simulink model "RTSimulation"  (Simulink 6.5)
settings: Solver=FixedStepDiscrete  StartTime=0.0  StopTime=inf  RelTol=1e-3
PreLoadFcn:
  | initialize
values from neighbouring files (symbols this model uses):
  actParams = [	bulkModulus   * pressCanon    [Copy of initialize.m]    (also in initialize.m = [bulkModulus	* pressCanon,)
  displFreq = inf    [initialize.m]
  flowCanon = 1.666667e+04    (= 16666.67)    [Copy of initialize.m]    (also in initialize.m)
  forceCanon = 1    [Copy of initialize.m]    (also in initialize.m)
  forceFreq = inf    [initialize.m]
  friction = 5			 				* 0.155000	 				* 0.00444822 				* area1    (= 2.71252900422)    [initialize.m]
  fsamp = 1 / samplePeriod    (= 1024)    [Copy of initialize.m]    (also in initialize.m; rampth.m = 1 / deltaT; randth.m = 1 / deltaT; rspect.m = 1.0 / tsamp)
  gasConstant = 1.8    [Copy of initialize.m]    (also in initialize.m)
  lengthCanon = 1    [Copy of initialize.m]    (also in initialize.m)
  massCanon = 1e-06    [Copy of initialize.m]    (also in initialize.m)
  maxDispl = ( (stroke2 + endLength2) * lengthCanon)'    [Copy of initialize.m]    (also in initialize.m = 576.2)
  maxOilVolume = volume * (1 - (precharge/supplyPress)^(1/gasConstant))    (= 211.391477114)    [Copy of initialize.m]    (also in initialize.m)
  maxVeloc = ( (maxFlow' * flowCanon ./ (area1 * areaCanon)) / velocCanon)'    [Copy of initialize.m]    (also in initialize.m = (maxFlow * flowCanon / (area1 * areaCanon)) / velocCanon; rampth.m = 2 * maxDispl / (nVeloc * deltaT))
  minDispl = (-(stroke1 + endLength1) * lengthCanon)'    [Copy of initialize.m]    (also in initialize.m = -576.2)
  minVeloc = (-(maxFlow' * flowCanon ./ (area2 * areaCanon)) / velocCanon)'    [Copy of initialize.m]    (also in initialize.m = -(maxFlow * flowCanon / (area2 * areaCanon)) / velocCanon)
  nAct = 5    [Copy of initialize.m]    (also in initialize.m = 1)
  nAdcU = 6    [Copy of initialize.m]    (also in initialize.m = 5)
  nDout = 4    [Copy of initialize.m]    (also in initialize.m)
  nDucU = 2    [Copy of initialize.m]    (also in initialize.m)
  nEncU = 3    [Copy of initialize.m]    (also in initialize.m)
  node = completenodestruct(node)    [Copy of initialize.m]    (also in initialize.m)
  precharge = 3000		 				* 6.894757e-03    (= 20.684271)    [Copy of initialize.m]    (also in initialize.m)
  pumpFlow = 1e20    (= 1e+20)    [Copy of initialize.m]    (also in initialize.m)
  returnPress = 3			 				* 0.1    (= 0.3)    [Copy of initialize.m]    (also in initialize.m)
  samplePeriod = controlPeriod/upsampleFactor    (= 0.0009765625)    [Copy of initialize.m]    (also in initialize.m; viewer.m = eval(getHeaderValue(header, 'DELTA_T')))
  springCanon = 1    [Copy of initialize.m]    (also in initialize.m)
  supplyPress = 280		 				* 0.1    (= 28)    [Copy of initialize.m]    (also in initialize.m)
  velocCanon = 1    [Copy of initialize.m]    (also in initialize.m)
  volume = 15.15		 				+ (  45		 				    * 2		 				   + 30		 				    * 6 )	 				* 5    (= 1365.15)    [Copy of initialize.m]    (also in initialize.m; quake.m = volume / 231.0)
  volumeCanon = 1e+06    (= 1000000)    [Copy of initialize.m]    (also in initialize.m)
  yieldDispl = 1.0    (= 1)    [initialize.m]
undefined symbols (not defined in the file or in its folder): DiscIntNeverNeededParam, dpforceFreq, mass, spring, staticForce
libraries: xpclib x5
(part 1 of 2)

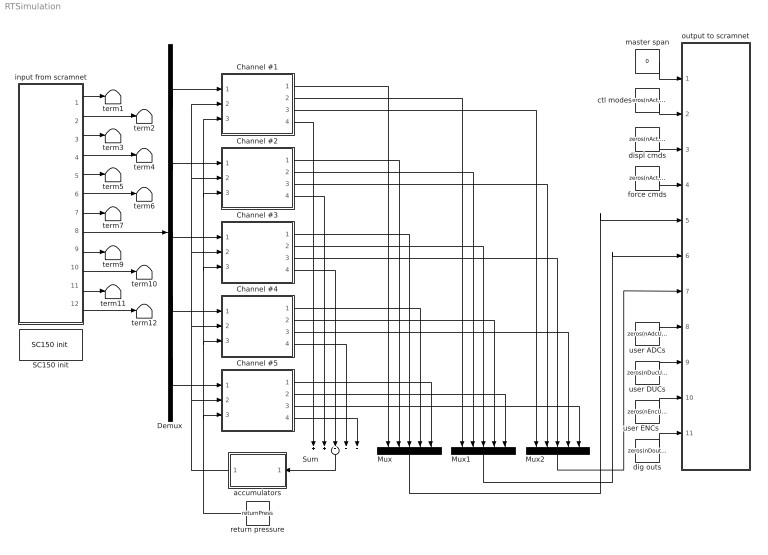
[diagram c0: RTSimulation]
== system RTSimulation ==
  Channel #1 : Subsystem  mask{id=1}
      mask prompts: id "Channel ID"
  Channel #2 : Subsystem  mask{id=2}
      mask prompts: id "Channel ID"
  Channel #3 : Subsystem  mask{id=3}
      mask prompts: id "Channel ID"
  Channel #4 : Subsystem  mask{id=4}
      mask prompts: id "Channel ID"
  Channel #5 : Subsystem  mask{id=5}
      mask prompts: id "Channel ID"
  Demux : Demux  Outputs=nAct
  Mux : Mux  Orientation=down  Inputs=nAct
  Mux1 : Mux  Orientation=down  Inputs=nAct
  Mux2 : Mux  Orientation=down  Inputs=nAct
  SC150 init : xpclib/Shared Memory/Systran/SC150 init   node=node  pci=-1
  Sum : Sum  Orientation=down  Inputs=+++++
  accumulators : Subsystem  Orientation=left
  ctl modes : Constant  Value=zeros(nAct, 1)  OutDataType=sfix(16)  ConRadixGroup=Use specified scaling  OutScaling=2^0  SampleTime=inf  FramePeriod=inf
  dig outs : Constant  Value=zeros(nDout, 1)  OutDataTypeMode=uint32  OutDataType=sfix(16)  ConRadixGroup=Use specified scaling  OutScaling=2^0  SampleTime=inf  FramePeriod=inf
  displ cmds : Constant  Value=zeros(nAct, 1)  OutDataType=sfix(16)  ConRadixGroup=Use specified scaling  OutScaling=2^0  SampleTime=inf  FramePeriod=inf
  force cmds : Constant  Value=zeros(nAct, 1)  OutDataType=sfix(16)  ConRadixGroup=Use specified scaling  OutScaling=2^0  SampleTime=inf  FramePeriod=inf
  input from scramnet : Subsystem
  master span : Constant  Value=0  OutDataType=sfix(16)  ConRadixGroup=Use specified scaling  OutScaling=2^0  SampleTime=inf  FramePeriod=inf
  output to scramnet : Subsystem
  return pressure : Constant  Orientation=left  Value=returnPress  OutDataType=sfix(16)  ConRadixGroup=Use specified scaling  OutScaling=2^0  SampleTime=inf  FramePeriod=inf
  term{1..7,9..12} (11 alike) : Terminator
  user ADCs : Constant  Value=zeros(nAdcU, 1)  OutDataType=sfix(16)  ConRadixGroup=Use specified scaling  OutScaling=2^0  SampleTime=inf  FramePeriod=inf
  user DUCs : Constant  Value=zeros(nDucU, 1)  OutDataType=sfix(16)  ConRadixGroup=Use specified scaling  OutScaling=2^0  SampleTime=inf  FramePeriod=inf
  user ENCs : Constant  Value=zeros(nEncU, 1)  OutDataType=sfix(16)  ConRadixGroup=Use specified scaling  OutScaling=2^0  SampleTime=inf  FramePeriod=inf
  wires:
  input from scramnet/6(force fbks) -> term6/1
  input from scramnet/10(user ducs) -> term10/1
  input from scramnet/12(dig inps) -> term12/1
  input from scramnet/4(force cmds) -> term4/1
  input from scramnet/5(displ fbks) -> term5/1
  input from scramnet/7(dpforce fbks) -> term7/1
  input from scramnet/9(user adcs) -> term9/1
  input from scramnet/11(user encs) -> term11/1
  input from scramnet/1(master span) -> term1/1
  input from scramnet/2(ctl modes) -> term2/1
  input from scramnet/3(displ cmds) -> term3/1
  master span/1 -> output to scramnet/1(master span)
  ctl modes/1 -> output to scramnet/2(ctl modes)
  displ cmds/1 -> output to scramnet/3(displ cmds)
  force cmds/1 -> output to scramnet/4(force cmds)
  user ADCs/1 -> output to scramnet/8(user adcs)
  user DUCs/1 -> output to scramnet/9(user ducs)
  user ENCs/1 -> output to scramnet/10(user encs)
  dig outs/1 -> output to scramnet/11(dig outs)
  Channel #1/4(flow) -> Sum/1
  Channel #2/4(flow) -> Sum/2
  Channel #3/4(flow) -> Sum/3
  Sum/1 -> accumulators/1(flow)
  Channel #4/4(flow) -> Sum/4
  Channel #5/4(flow) -> Sum/5
  Channel #1/1(displ) -> Mux/1
  Channel #2/1(displ) -> Mux/2
  Channel #3/1(displ) -> Mux/3
  Channel #4/1(displ) -> Mux/4
  Channel #5/1(displ) -> Mux/5
  Channel #1/2(force) -> Mux1/1
  Channel #2/2(force) -> Mux1/2
  Channel #3/2(force) -> Mux1/3
  Channel #4/2(force) -> Mux1/4
  Channel #5/2(force) -> Mux1/5
  Channel #1/3(dpforce) -> Mux2/1
  Channel #2/3(dpforce) -> Mux2/2
  Channel #3/3(dpforce) -> Mux2/3
  Channel #4/3(dpforce) -> Mux2/4
  Channel #5/3(dpforce) -> Mux2/5
  Mux/1 -> output to scramnet/5(displ fbks)
  Mux1/1 -> output to scramnet/6(force fbks)
  Mux2/1 -> output to scramnet/7(dpforce fbks)
  input from scramnet/8(valve cmds) -> Demux/1
  Demux/1 -> Channel #1/1(valve cmd)
  Demux/2 -> Channel #2/1(valve cmd)
  Demux/3 -> Channel #3/1(valve cmd)
  Demux/4 -> Channel #4/1(valve cmd)
  Demux/5 -> Channel #5/1(valve cmd)
  accumulators/1(press) -> Channel #2/2(spl press), Channel #1/2(spl press), Channel #3/2(spl press), Channel #4/2(spl press), Channel #5/2(spl press)
  return pressure/1 -> Channel #2/3(rtn press), Channel #1/3(rtn press), Channel #3/3(rtn press), Channel #4/3(rtn press), Channel #5/3(rtn press)

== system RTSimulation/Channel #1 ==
  valve cmd : Inport
  spl press : Inport  Port=2
  rtn press : Inport  Port=3
  displ cond filter : Subsystem  mask{freq3dB=displFreq(id), fsamp=fsamp}
      mask prompts: freq3dB "3 dB cutoff frequency (inf, 500, 300, 100, 50 Hz)"; fsamp "Sampling frequency (Hz)"
      mask init:
      | if isempty(freq3dB)
      | 	freq3dB = fsamp;
      | elseif freq3dB == 500
      | 	freq3dB = 485;
      | elseif freq3dB == 300
      | 	freq3dB = 204.9;
      | elseif freq3dB == 100
      | 	freq3dB = 56.5;
      | elseif freq3dB == 50
      | 	freq3dB = 27.8;
      | else
      | 	freq3dB = fsamp;
      | end
      | if freq3dB > fsamp/2
      | 	a = [1];
      | 	b = [1];
      | else
      | 	[b, a] = ellip(4, 0.001, 60.0, 2*freq3dB/fsamp);
      | end
  dpforce cond filter : Subsystem  mask{freq3dB=dpforceFreq(id), fsamp=fsamp}
      mask prompts: freq3dB "3 dB cutoff frequency (inf, 500, 300, 100, 50 Hz)"; fsamp "Sampling frequency (Hz)"
      mask init:
      | if isempty(freq3dB)
      | 	freq3dB = fsamp;
      | elseif freq3dB == 500
      | 	freq3dB = 485;
      | elseif freq3dB == 300
      | 	freq3dB = 204.9;
      | elseif freq3dB == 100
      | 	freq3dB = 56.5;
      | elseif freq3dB == 50
      | 	freq3dB = 27.8;
      | else
      | 	freq3dB = fsamp;
      | end
      | if freq3dB > fsamp/2
      | 	a = [1];
      | 	b = [1];
      | else
      | 	[b, a] = ellip(4, 0.001, 60.0, 2*freq3dB/fsamp);
      | end
  force cond filter : Subsystem  mask{freq3dB=forceFreq((id)), fsamp=fsamp}
      mask prompts: freq3dB "3 dB cutoff frequency (inf, 500, 300, 100, 50 Hz)"; fsamp "Sampling frequency (Hz)"
      mask init:
      | if isempty(freq3dB)
      | 	freq3dB = fsamp;
      | elseif freq3dB == 500
      | 	freq3dB = 485;
      | elseif freq3dB == 300
      | 	freq3dB = 204.9;
      | elseif freq3dB == 100
      | 	freq3dB = 56.5;
      | elseif freq3dB == 50
      | 	freq3dB = 27.8;
      | else
      | 	freq3dB = fsamp;
      | end
      | if freq3dB > fsamp/2
      | 	a = [1];
      | 	b = [1];
      | else
      | 	[b, a] = ellip(4, 0.001, 60.0, 2*freq3dB/fsamp);
      | end
  payload : Subsystem
  servovalve & actuator : Subsystem  mask(Actuator){params=actParams(:,id)}
      mask prompts: params "Parameter vector"
  displ : Outport
  force : Outport  Port=2
  dpforce : Outport  Port=3
  flow : Outport  Port=4
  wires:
  dpforce cond filter/1(out) -> dpforce/1
  force cond filter/1(out) -> force/1
  displ cond filter/1(out) -> displ/1
  servovalve & actuator/1(force) -> payload/1(force), dpforce cond filter/1(inp), force cond filter/1(inp)
  servovalve & actuator/2(flow) -> flow/1
  spl press/1 -> servovalve & actuator/4(spl press)
  rtn press/1 -> servovalve & actuator/5(rtn press)
  valve cmd/1 -> servovalve & actuator/1(cmd)
  payload/1(displ) -> servovalve & actuator/2(displ), displ cond filter/1(inp)
  payload/2(veloc) -> servovalve & actuator/3(veloc)

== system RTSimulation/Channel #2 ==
  valve cmd : Inport
  spl press : Inport  Port=2
  rtn press : Inport  Port=3
  displ cond filter : Subsystem  mask{freq3dB=displFreq(id), fsamp=fsamp}
      mask prompts: freq3dB "3 dB cutoff frequency (inf, 500, 300, 100, 50 Hz)"; fsamp "Sampling frequency (Hz)"
      mask init:
      | if isempty(freq3dB)
      | 	freq3dB = fsamp;
      | elseif freq3dB == 500
      | 	freq3dB = 485;
      | elseif freq3dB == 300
      | 	freq3dB = 204.9;
      | elseif freq3dB == 100
      | 	freq3dB = 56.5;
      | elseif freq3dB == 50
      | 	freq3dB = 27.8;
      | else
      | 	freq3dB = fsamp;
      | end
      | if freq3dB > fsamp/2
      | 	a = [1];
      | 	b = [1];
      | else
      | 	[b, a] = ellip(4, 0.001, 60.0, 2*freq3dB/fsamp);
      | end
  dpforce cond filter : Subsystem  mask{freq3dB=dpforceFreq(id), fsamp=fsamp}
      mask prompts: freq3dB "3 dB cutoff frequency (inf, 500, 300, 100, 50 Hz)"; fsamp "Sampling frequency (Hz)"
      mask init:
      | if isempty(freq3dB)
      | 	freq3dB = fsamp;
      | elseif freq3dB == 500
      | 	freq3dB = 485;
      | elseif freq3dB == 300
      | 	freq3dB = 204.9;
      | elseif freq3dB == 100
      | 	freq3dB = 56.5;
      | elseif freq3dB == 50
      | 	freq3dB = 27.8;
      | else
      | 	freq3dB = fsamp;
      | end
      | if freq3dB > fsamp/2
      | 	a = [1];
      | 	b = [1];
      | else
      | 	[b, a] = ellip(4, 0.001, 60.0, 2*freq3dB/fsamp);
      | end
  force cond filter : Subsystem  mask{freq3dB=forceFreq((id)), fsamp=fsamp}
      mask prompts: freq3dB "3 dB cutoff frequency (inf, 500, 300, 100, 50 Hz)"; fsamp "Sampling frequency (Hz)"
      mask init:
      | if isempty(freq3dB)
      | 	freq3dB = fsamp;
      | elseif freq3dB == 500
      | 	freq3dB = 485;
      | elseif freq3dB == 300
      | 	freq3dB = 204.9;
      | elseif freq3dB == 100
      | 	freq3dB = 56.5;
      | elseif freq3dB == 50
      | 	freq3dB = 27.8;
      | else
      | 	freq3dB = fsamp;
      | end
      | if freq3dB > fsamp/2
      | 	a = [1];
      | 	b = [1];
      | else
      | 	[b, a] = ellip(4, 0.001, 60.0, 2*freq3dB/fsamp);
      | end
  payload : Subsystem
  servovalve & actuator : Subsystem  mask(Actuator){params=actParams(:,id)}
      mask prompts: params "Parameter vector"
  displ : Outport
  force : Outport  Port=2
  dpforce : Outport  Port=3
  flow : Outport  Port=4
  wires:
  payload/2(veloc) -> servovalve & actuator/3(veloc)
  payload/1(displ) -> displ cond filter/1(inp), servovalve & actuator/2(displ)
  valve cmd/1 -> servovalve & actuator/1(cmd)
  rtn press/1 -> servovalve & actuator/5(rtn press)
  spl press/1 -> servovalve & actuator/4(spl press)
  servovalve & actuator/2(flow) -> flow/1
  servovalve & actuator/1(force) -> force cond filter/1(inp), dpforce cond filter/1(inp), payload/1(force)
  displ cond filter/1(out) -> displ/1
  force cond filter/1(out) -> force/1
  dpforce cond filter/1(out) -> dpforce/1

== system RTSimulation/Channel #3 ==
  valve cmd : Inport
  spl press : Inport  Port=2
  rtn press : Inport  Port=3
  displ cond filter : Subsystem  mask{freq3dB=displFreq(id), fsamp=fsamp}
      mask prompts: freq3dB "3 dB cutoff frequency (inf, 500, 300, 100, 50 Hz)"; fsamp "Sampling frequency (Hz)"
      mask init:
      | if isempty(freq3dB)
      | 	freq3dB = fsamp;
      | elseif freq3dB == 500
      | 	freq3dB = 485;
      | elseif freq3dB == 300
      | 	freq3dB = 204.9;
      | elseif freq3dB == 100
      | 	freq3dB = 56.5;
      | elseif freq3dB == 50
      | 	freq3dB = 27.8;
      | else
      | 	freq3dB = fsamp;
      | end
      | if freq3dB > fsamp/2
      | 	a = [1];
      | 	b = [1];
      | else
      | 	[b, a] = ellip(4, 0.001, 60.0, 2*freq3dB/fsamp);
      | end
  dpforce cond filter : Subsystem  mask{freq3dB=dpforceFreq(id), fsamp=fsamp}
      mask prompts: freq3dB "3 dB cutoff frequency (inf, 500, 300, 100, 50 Hz)"; fsamp "Sampling frequency (Hz)"
      mask init:
      | if isempty(freq3dB)
      | 	freq3dB = fsamp;
      | elseif freq3dB == 500
      | 	freq3dB = 485;
      | elseif freq3dB == 300
      | 	freq3dB = 204.9;
      | elseif freq3dB == 100
      | 	freq3dB = 56.5;
      | elseif freq3dB == 50
      | 	freq3dB = 27.8;
      | else
      | 	freq3dB = fsamp;
      | end
      | if freq3dB > fsamp/2
      | 	a = [1];
      | 	b = [1];
      | else
      | 	[b, a] = ellip(4, 0.001, 60.0, 2*freq3dB/fsamp);
      | end
  force cond filter : Subsystem  mask{freq3dB=forceFreq((id)), fsamp=fsamp}
      mask prompts: freq3dB "3 dB cutoff frequency (inf, 500, 300, 100, 50 Hz)"; fsamp "Sampling frequency (Hz)"
      mask init:
      | if isempty(freq3dB)
      | 	freq3dB = fsamp;
      | elseif freq3dB == 500
      | 	freq3dB = 485;
      | elseif freq3dB == 300
      | 	freq3dB = 204.9;
      | elseif freq3dB == 100
      | 	freq3dB = 56.5;
      | elseif freq3dB == 50
      | 	freq3dB = 27.8;
      | else
      | 	freq3dB = fsamp;
      | end
      | if freq3dB > fsamp/2
      | 	a = [1];
      | 	b = [1];
      | else
      | 	[b, a] = ellip(4, 0.001, 60.0, 2*freq3dB/fsamp);
      | end
  payload : Subsystem
  servovalve & actuator : Subsystem  mask(Actuator){params=actParams(:,id)}
      mask prompts: params "Parameter vector"
  displ : Outport
  force : Outport  Port=2
  dpforce : Outport  Port=3
  flow : Outport  Port=4
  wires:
  dpforce cond filter/1(out) -> dpforce/1
  force cond filter/1(out) -> force/1
  displ cond filter/1(out) -> displ/1
  servovalve & actuator/1(force) -> payload/1(force), dpforce cond filter/1(inp), force cond filter/1(inp)
  servovalve & actuator/2(flow) -> flow/1
  spl press/1 -> servovalve & actuator/4(spl press)
  rtn press/1 -> servovalve & actuator/5(rtn press)
  valve cmd/1 -> servovalve & actuator/1(cmd)
  payload/1(displ) -> servovalve & actuator/2(displ), displ cond filter/1(inp)
  payload/2(veloc) -> servovalve & actuator/3(veloc)

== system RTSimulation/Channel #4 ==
  valve cmd : Inport
  spl press : Inport  Port=2
  rtn press : Inport  Port=3
  displ cond filter : Subsystem  mask{freq3dB=displFreq(id), fsamp=fsamp}
      mask prompts: freq3dB "3 dB cutoff frequency (inf, 500, 300, 100, 50 Hz)"; fsamp "Sampling frequency (Hz)"
      mask init:
      | if isempty(freq3dB)
      | 	freq3dB = fsamp;
      | elseif freq3dB == 500
      | 	freq3dB = 485;
      | elseif freq3dB == 300
      | 	freq3dB = 204.9;
      | elseif freq3dB == 100
      | 	freq3dB = 56.5;
      | elseif freq3dB == 50
      | 	freq3dB = 27.8;
      | else
      | 	freq3dB = fsamp;
      | end
      | if freq3dB > fsamp/2
      | 	a = [1];
      | 	b = [1];
      | else
      | 	[b, a] = ellip(4, 0.001, 60.0, 2*freq3dB/fsamp);
      | end
  dpforce cond filter : Subsystem  mask{freq3dB=dpforceFreq(id), fsamp=fsamp}
      mask prompts: freq3dB "3 dB cutoff frequency (inf, 500, 300, 100, 50 Hz)"; fsamp "Sampling frequency (Hz)"
      mask init:
      | if isempty(freq3dB)
      | 	freq3dB = fsamp;
      | elseif freq3dB == 500
      | 	freq3dB = 485;
      | elseif freq3dB == 300
      | 	freq3dB = 204.9;
      | elseif freq3dB == 100
      | 	freq3dB = 56.5;
      | elseif freq3dB == 50
      | 	freq3dB = 27.8;
      | else
      | 	freq3dB = fsamp;
      | end
      | if freq3dB > fsamp/2
      | 	a = [1];
      | 	b = [1];
      | else
      | 	[b, a] = ellip(4, 0.001, 60.0, 2*freq3dB/fsamp);
      | end
  force cond filter : Subsystem  mask{freq3dB=forceFreq((id)), fsamp=fsamp}
      mask prompts: freq3dB "3 dB cutoff frequency (inf, 500, 300, 100, 50 Hz)"; fsamp "Sampling frequency (Hz)"
      mask init:
      | if isempty(freq3dB)
      | 	freq3dB = fsamp;
      | elseif freq3dB == 500
      | 	freq3dB = 485;
      | elseif freq3dB == 300
      | 	freq3dB = 204.9;
      | elseif freq3dB == 100
      | 	freq3dB = 56.5;
      | elseif freq3dB == 50
      | 	freq3dB = 27.8;
      | else
      | 	freq3dB = fsamp;
      | end
      | if freq3dB > fsamp/2
      | 	a = [1];
      | 	b = [1];
      | else
      | 	[b, a] = ellip(4, 0.001, 60.0, 2*freq3dB/fsamp);
      | end
  payload : Subsystem
  servovalve & actuator : Subsystem  mask(Actuator){params=actParams(:,id)}
      mask prompts: params "Parameter vector"
  displ : Outport
  force : Outport  Port=2
  dpforce : Outport  Port=3
  flow : Outport  Port=4
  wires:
  payload/2(veloc) -> servovalve & actuator/3(veloc)
  payload/1(displ) -> displ cond filter/1(inp), servovalve & actuator/2(displ)
  valve cmd/1 -> servovalve & actuator/1(cmd)
  rtn press/1 -> servovalve & actuator/5(rtn press)
  spl press/1 -> servovalve & actuator/4(spl press)
  servovalve & actuator/2(flow) -> flow/1
  servovalve & actuator/1(force) -> force cond filter/1(inp), dpforce cond filter/1(inp), payload/1(force)
  displ cond filter/1(out) -> displ/1
  force cond filter/1(out) -> force/1
  dpforce cond filter/1(out) -> dpforce/1

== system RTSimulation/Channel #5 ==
  valve cmd : Inport
  spl press : Inport  Port=2
  rtn press : Inport  Port=3
  displ cond filter : Subsystem  mask{freq3dB=displFreq(id), fsamp=fsamp}
      mask prompts: freq3dB "3 dB cutoff frequency (inf, 500, 300, 100, 50 Hz)"; fsamp "Sampling frequency (Hz)"
      mask init:
      | if isempty(freq3dB)
      | 	freq3dB = fsamp;
      | elseif freq3dB == 500
      | 	freq3dB = 485;
      | elseif freq3dB == 300
      | 	freq3dB = 204.9;
      | elseif freq3dB == 100
      | 	freq3dB = 56.5;
      | elseif freq3dB == 50
      | 	freq3dB = 27.8;
      | else
      | 	freq3dB = fsamp;
      | end
      | if freq3dB > fsamp/2
      | 	a = [1];
      | 	b = [1];
      | else
      | 	[b, a] = ellip(4, 0.001, 60.0, 2*freq3dB/fsamp);
      | end
  dpforce cond filter : Subsystem  mask{freq3dB=dpforceFreq(id), fsamp=fsamp}
      mask prompts: freq3dB "3 dB cutoff frequency (inf, 500, 300, 100, 50 Hz)"; fsamp "Sampling frequency (Hz)"
      mask init:
      | if isempty(freq3dB)
      | 	freq3dB = fsamp;
      | elseif freq3dB == 500
      | 	freq3dB = 485;
      | elseif freq3dB == 300
      | 	freq3dB = 204.9;
      | elseif freq3dB == 100
      | 	freq3dB = 56.5;
      | elseif freq3dB == 50
      | 	freq3dB = 27.8;
      | else
      | 	freq3dB = fsamp;
      | end
      | if freq3dB > fsamp/2
      | 	a = [1];
      | 	b = [1];
      | else
      | 	[b, a] = ellip(4, 0.001, 60.0, 2*freq3dB/fsamp);
      | end
  force cond filter : Subsystem  mask{freq3dB=forceFreq((id)), fsamp=fsamp}
      mask prompts: freq3dB "3 dB cutoff frequency (inf, 500, 300, 100, 50 Hz)"; fsamp "Sampling frequency (Hz)"
      mask init:
      | if isempty(freq3dB)
      | 	freq3dB = fsamp;
      | elseif freq3dB == 500
      | 	freq3dB = 485;
      | elseif freq3dB == 300
      | 	freq3dB = 204.9;
      | elseif freq3dB == 100
      | 	freq3dB = 56.5;
      | elseif freq3dB == 50
      | 	freq3dB = 27.8;
      | else
      | 	freq3dB = fsamp;
      | end
      | if freq3dB > fsamp/2
      | 	a = [1];
      | 	b = [1];
      | else
      | 	[b, a] = ellip(4, 0.001, 60.0, 2*freq3dB/fsamp);
      | end
  payload : Subsystem
  servovalve & actuator : Subsystem  mask(Actuator){params=actParams(:,id)}
      mask prompts: params "Parameter vector"
  displ : Outport
  force : Outport  Port=2
  dpforce : Outport  Port=3
  flow : Outport  Port=4
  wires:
  dpforce cond filter/1(out) -> dpforce/1
  force cond filter/1(out) -> force/1
  displ cond filter/1(out) -> displ/1
  servovalve & actuator/1(force) -> payload/1(force), dpforce cond filter/1(inp), force cond filter/1(inp)
  servovalve & actuator/2(flow) -> flow/1
  spl press/1 -> servovalve & actuator/4(spl press)
  rtn press/1 -> servovalve & actuator/5(rtn press)
  valve cmd/1 -> servovalve & actuator/1(cmd)
  payload/1(displ) -> servovalve & actuator/2(displ), displ cond filter/1(inp)
  payload/2(veloc) -> servovalve & actuator/3(veloc)

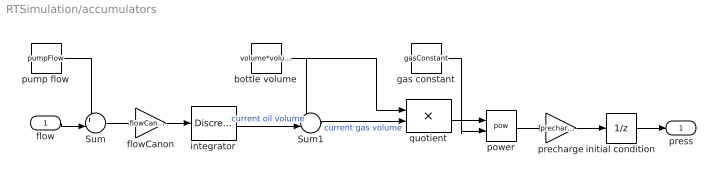
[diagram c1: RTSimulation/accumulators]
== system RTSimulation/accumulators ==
  flow : Inport
  Sum : Sum  Inputs=+-|
  Sum1 : Sum  Inputs=+-|
  bottle volume : Constant  Value=volume*volumeCanon  OutDataType=sfix(16)  ConRadixGroup=Use specified scaling  OutScaling=2^0  SampleTime=inf  FramePeriod=inf
  flowCanon : Gain  Gain=flowCanon
  gas constant : Constant  Value=gasConstant  OutDataType=sfix(16)  ConRadixGroup=Use specified scaling  OutScaling=2^0  SampleTime=inf  FramePeriod=inf
  initial condition : UnitDelay  X0=supplyPress  SampleTime=-1
  integrator : DiscreteIntegrator  InitialCondition=maxOilVolume*volumeCanon  SampleTime=-1  LimitOutput=on  UpperSaturationLimit=maxOilVolume*volumeCanon  LowerSaturationLimit=0  ICPrevOutput=DiscIntNeverNeededParam  ICPrevScaledInput=DiscIntNeverNeededParam
  power : Math  Operator=pow
  precharge : Gain  Gain=precharge
  pump flow : Constant  Value=pumpFlow  OutDataType=sfix(16)  ConRadixGroup=Use specified scaling  OutScaling=2^0  SampleTime=inf  FramePeriod=inf
  quotient : Product  Inputs=*/
  press : Outport
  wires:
  pump flow/1 -> Sum/1
  Sum/1 -> flowCanon/1
  bottle volume/1 -> Sum1/1, quotient/1
  gas constant/1 -> power/2
  power/1 -> precharge/1
  precharge/1 -> initial condition/1
  Sum1/1 -> quotient/2  "current gas volume"
  quotient/1 -> power/1
  integrator/1 -> Sum1/2  "current oil volume"
  flow/1 -> Sum/2
  flowCanon/1 -> integrator/1
  initial condition/1 -> press/1

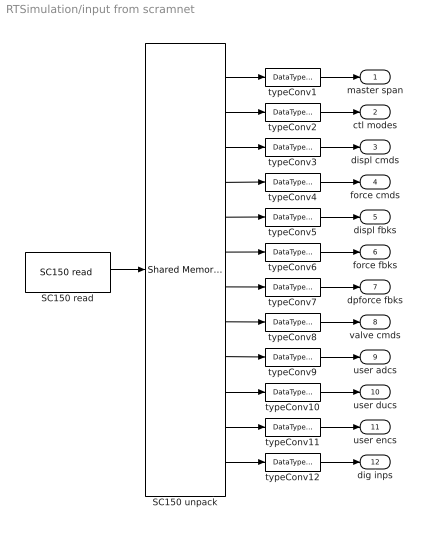
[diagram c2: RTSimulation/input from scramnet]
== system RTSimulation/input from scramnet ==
  SC150 read : xpclib/Shared Memory/Systran/SC150 read   partition=node.Partitions(12:23)  ts=samplePeriod  pci=-1
  SC150 unpack : xpclib/Shared Memory/Shared Memory Unpack   partition=node.Partitions(12:23)
  typeConv{1,3..11} (10 alike) : DataTypeConversion  OutDataTypeMode=double
  typeConv12 : DataTypeConversion  OutDataTypeMode=uint32
  typeConv2 : DataTypeConversion  OutDataTypeMode=uint32
  master span : Outport
  ctl modes : Outport  Port=2
  displ cmds : Outport  Port=3
  force cmds : Outport  Port=4
  displ fbks : Outport  Port=5
  force fbks : Outport  Port=6
  dpforce fbks : Outport  Port=7
  valve cmds : Outport  Port=8
  user adcs : Outport  Port=9
  user ducs : Outport  Port=10
  user encs : Outport  Port=11
  dig inps : Outport  Port=12
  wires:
  typeConv11/1 -> user encs/1
  typeConv10/1 -> user ducs/1
  typeConv12/1 -> dig inps/1
  typeConv9/1 -> user adcs/1
  typeConv8/1 -> valve cmds/1
  typeConv7/1 -> dpforce fbks/1
  typeConv6/1 -> force fbks/1
  typeConv5/1 -> displ fbks/1
  typeConv4/1 -> force cmds/1
  typeConv3/1 -> displ cmds/1
  typeConv1/1 -> master span/1
  SC150 read/1 -> SC150 unpack/1
  typeConv2/1 -> ctl modes/1
  SC150 unpack/1 -> typeConv1/1
  SC150 unpack/2 -> typeConv2/1
  SC150 unpack/3 -> typeConv3/1
  SC150 unpack/4 -> typeConv4/1
  SC150 unpack/5 -> typeConv5/1
  SC150 unpack/6 -> typeConv6/1
  SC150 unpack/7 -> typeConv7/1
  SC150 unpack/8 -> typeConv8/1
  SC150 unpack/9 -> typeConv9/1
  SC150 unpack/10 -> typeConv10/1
  SC150 unpack/11 -> typeConv11/1
  SC150 unpack/12 -> typeConv12/1

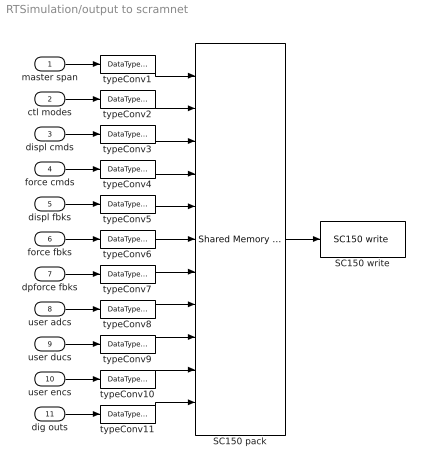
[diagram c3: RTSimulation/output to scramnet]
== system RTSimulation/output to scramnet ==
  master span : Inport
  ctl modes : Inport  Port=2
  displ cmds : Inport  Port=3
  force cmds : Inport  Port=4
  displ fbks : Inport  Port=5
  force fbks : Inport  Port=6
  dpforce fbks : Inport  Port=7
  user adcs : Inport  Port=8
  user ducs : Inport  Port=9
  user encs : Inport  Port=10
  dig outs : Inport  Port=11
  SC150 pack : xpclib/Shared Memory/Shared Memory Pack   partition=node.Partitions(1:11)
  SC150 write : xpclib/Shared Memory/Systran/SC150 write   partition=node.Partitions(1:11)  ts=samplePeriod  pci=-1
  typeConv{1,3..10} (9 alike) : DataTypeConversion  OutDataTypeMode=single
  typeConv11 : DataTypeConversion  OutDataTypeMode=uint32
  typeConv2 : DataTypeConversion  OutDataTypeMode=uint32
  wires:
  typeConv11/1 -> SC150 pack/11
  typeConv10/1 -> SC150 pack/10
  typeConv9/1 -> SC150 pack/9
  typeConv8/1 -> SC150 pack/8
  typeConv7/1 -> SC150 pack/7
  typeConv6/1 -> SC150 pack/6
  typeConv5/1 -> SC150 pack/5
  dig outs/1 -> typeConv11/1
  user encs/1 -> typeConv10/1
  user ducs/1 -> typeConv9/1
  user adcs/1 -> typeConv8/1
  dpforce fbks/1 -> typeConv7/1
  force fbks/1 -> typeConv6/1
  displ fbks/1 -> typeConv5/1
  force cmds/1 -> typeConv4/1
  master span/1 -> typeConv1/1
  SC150 pack/1 -> SC150 write/1
  displ cmds/1 -> typeConv3/1
  ctl modes/1 -> typeConv2/1
  typeConv1/1 -> SC150 pack/1
  typeConv2/1 -> SC150 pack/2
  typeConv3/1 -> SC150 pack/3
  typeConv4/1 -> SC150 pack/4

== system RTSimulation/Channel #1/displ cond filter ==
  inp : Inport
  filter : DiscreteFilter  Numerator=b  Denominator=a  SampleTime=-1
  out : Outport
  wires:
  filter/1 -> out/1
  inp/1 -> filter/1

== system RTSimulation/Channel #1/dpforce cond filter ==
  inp : Inport
  filter : DiscreteFilter  Numerator=b  Denominator=a  SampleTime=-1
  out : Outport
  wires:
  inp/1 -> filter/1
  filter/1 -> out/1

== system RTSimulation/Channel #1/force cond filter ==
  inp : Inport
  filter : DiscreteFilter  Numerator=b  Denominator=a  SampleTime=-1
  out : Outport
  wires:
  filter/1 -> out/1
  inp/1 -> filter/1

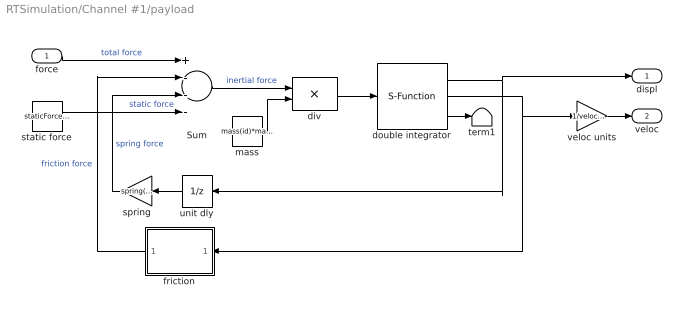
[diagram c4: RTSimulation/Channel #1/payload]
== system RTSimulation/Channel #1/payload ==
  force : Inport
  Sum : Sum  Inputs=+---
  div : Product  Inputs=*/
  double integrator : S-Function  FunctionName=doubleintegrator  Parameters=maxDispl, minDispl, initDispl, maxVeloc, minVeloc, initVeloc, samplePeriod  mask(Double integrator){maxDispl=maxDispl(id), minDispl=minDispl(id), initDispl=0, maxVeloc=maxVeloc(id)*velocCanon, minVeloc=minVeloc(id)*velocCanon, initVeloc=0, samplePeriod=samplePeriod}
      mask prompts: maxDispl "Maximum displacement"; minDispl "Minimum displacement"; initDispl "Initial displacement"; maxVeloc "Maximum velocity"; minVeloc "Minimum velocity"; initVeloc "Initial velocity"; samplePeriod "Sample period (sec)"
      mask help: Integrates acceleration twice to produce velocity and displacement. When clipping occurs, acceleration, velocity and displacement are adjusted accordingly.
  friction : Subsystem  Orientation=left  mask{friction=friction(id)*forceCanon, yieldDispl=yieldDispl(id)*lengthCanon, hysteresis=0}
      mask prompts: friction "Sliding friction"; yieldDispl "Equiv. yield displacement (in)"; hysteresis "Hysteresis constant"
  mass : Constant  Value=mass(id)*massCanon  OutDataType=sfix(16)  ConRadixGroup=Use specified scaling  OutScaling=2^0  SampleTime=inf  FramePeriod=inf
  spring : Gain  Orientation=left  Gain=spring(id)*springCanon
  static force : Constant  Value=staticForce(id)*forceCanon  OutDataType=sfix(16)  ConRadixGroup=Use specified scaling  OutScaling=2^0  SampleTime=inf  FramePeriod=inf
  term1 : Terminator
  unit dly : UnitDelay  Orientation=left  SampleTime=-1
  veloc units : Gain  Gain=1/velocCanon
  displ : Outport
  veloc : Outport  Port=2
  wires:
  double integrator/2 -> friction/1(veloc), veloc units/1
  double integrator/1 -> unit dly/1, displ/1
  div/1 -> double integrator/1
  double integrator/3 -> term1/1
  spring/1 -> Sum/3  "spring force"
  mass/1 -> div/2
  force/1 -> Sum/1  "total force"
  static force/1 -> Sum/4  "static force"
  Sum/1 -> div/1  "inertial force"
  veloc units/1 -> veloc/1
  unit dly/1 -> spring/1
  friction/1(force) -> Sum/2  "friction force"

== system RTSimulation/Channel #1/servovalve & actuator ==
  note: Parameter vector: 1: oil bulk modulus (force/displ^2) 2: servovalve delay (sec) 3: servovalve overlap 4: rated pressure (force/displ^2) 5: rated flow at rated pressure (displ^3/sec) 6: nominal flow at rated pressure (displ^3/sec) 7: actuator piston area 1 (displ^2) 8: actuator piston area 2 (displ^2) 9: actuator usable stroke 1 (displ) 10: actuator usable stroke 2 (displ) 11: actuator end cushion length 1 (displ) 12: actuator end cushion length 2 (displ) 13: additional port volume 1 (displ^3) 14: additional port volume 1 (displ^3) 15: actuator parasitic damping factor 16: cross-chamber leakage factor (flow/press) 17: ratio port openings according to area 18: sample period (sec) Conversion factors used for converting signals from external (user) to internal (canonical) units: 19: displacement 20: velocity 21: force 22: pressure 23: flow
  note: Note: "1" and "2" denote actuator cylinders on either side of the actuator piston. With positive valve drive, oil is ported into cylinder 1, resulting in positive displacement.
  note: Auxiliary diagnostic output vector: 1: valve opening 2: C1 pressure 3: C2 pressure 4: delta pressure 5: force 6: velocity 7: C1 flow 8: C2 flow 9: total flow 10: kinematic flow 11: compressibility flow 12: leakage flow 13: C1 oilspring displacement 14: C2 oilspring displacement 15: C1 oilspring velocity 16: C2 oilspring velocity
  cmd : Inport
  displ : Inport  Port=2
  veloc : Inport  Port=3
  spl press : Inport  Port=4
  rtn press : Inport  Port=5
  abs : Abs  SaturateOnIntegerOverflow=on  SampleTime=-1
  actuator : S-Function  FunctionName=Actuator  Parameters=params
  total flow sel : Selector  InputType=Vector  ElementSrc=Internal  Elements=9  RowSrc=Internal  Rows=1  ColumnSrc=Internal  Columns=1  IndexIsStartValue=off
  force : Outport
  flow : Outport  Port=2
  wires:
  spl press/1 -> actuator/4
  rtn press/1 -> actuator/5
  cmd/1 -> actuator/1
  actuator/1 -> force/1
  displ/1 -> actuator/2
  veloc/1 -> actuator/3
  actuator/2 -> total flow sel/1
  total flow sel/1 -> abs/1
  abs/1 -> flow/1

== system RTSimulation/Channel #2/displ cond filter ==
  inp : Inport
  filter : DiscreteFilter  Numerator=b  Denominator=a  SampleTime=-1
  out : Outport
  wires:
  inp/1 -> filter/1
  filter/1 -> out/1

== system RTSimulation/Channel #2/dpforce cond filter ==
  inp : Inport
  filter : DiscreteFilter  Numerator=b  Denominator=a  SampleTime=-1
  out : Outport
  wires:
  filter/1 -> out/1
  inp/1 -> filter/1

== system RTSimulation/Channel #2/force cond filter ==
  inp : Inport
  filter : DiscreteFilter  Numerator=b  Denominator=a  SampleTime=-1
  out : Outport
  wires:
  inp/1 -> filter/1
  filter/1 -> out/1

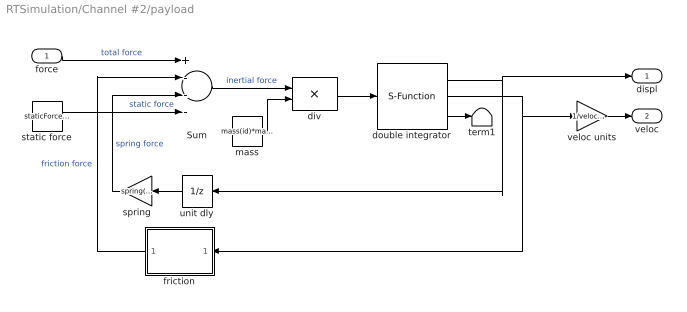
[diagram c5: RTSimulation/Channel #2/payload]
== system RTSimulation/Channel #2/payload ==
  force : Inport
  Sum : Sum  Inputs=+---
  div : Product  Inputs=*/
  double integrator : S-Function  FunctionName=doubleintegrator  Parameters=maxDispl, minDispl, initDispl, maxVeloc, minVeloc, initVeloc, samplePeriod  mask(Double integrator){maxDispl=maxDispl(id), minDispl=minDispl(id), initDispl=0, maxVeloc=maxVeloc(id)*velocCanon, minVeloc=minVeloc(id)*velocCanon, initVeloc=0, samplePeriod=samplePeriod}
      mask prompts: maxDispl "Maximum displacement"; minDispl "Minimum displacement"; initDispl "Initial displacement"; maxVeloc "Maximum velocity"; minVeloc "Minimum velocity"; initVeloc "Initial velocity"; samplePeriod "Sample period (sec)"
      mask help: Integrates acceleration twice to produce velocity and displacement. When clipping occurs, acceleration, velocity and displacement are adjusted accordingly.
  friction : Subsystem  Orientation=left  mask{friction=friction(id)*forceCanon, yieldDispl=yieldDispl(id)*lengthCanon, hysteresis=0}
      mask prompts: friction "Sliding friction"; yieldDispl "Equiv. yield displacement (in)"; hysteresis "Hysteresis constant"
  mass : Constant  Value=mass(id)*massCanon  OutDataType=sfix(16)  ConRadixGroup=Use specified scaling  OutScaling=2^0  SampleTime=inf  FramePeriod=inf
  spring : Gain  Orientation=left  Gain=spring(id)*springCanon
  static force : Constant  Value=staticForce(id)*forceCanon  OutDataType=sfix(16)  ConRadixGroup=Use specified scaling  OutScaling=2^0  SampleTime=inf  FramePeriod=inf
  term1 : Terminator
  unit dly : UnitDelay  Orientation=left  SampleTime=-1
  veloc units : Gain  Gain=1/velocCanon
  displ : Outport
  veloc : Outport  Port=2
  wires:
  friction/1(force) -> Sum/2  "friction force"
  unit dly/1 -> spring/1
  veloc units/1 -> veloc/1
  Sum/1 -> div/1  "inertial force"
  static force/1 -> Sum/4  "static force"
  force/1 -> Sum/1  "total force"
  mass/1 -> div/2
  spring/1 -> Sum/3  "spring force"
  double integrator/3 -> term1/1
  div/1 -> double integrator/1
  double integrator/1 -> displ/1, unit dly/1
  double integrator/2 -> veloc units/1, friction/1(veloc)

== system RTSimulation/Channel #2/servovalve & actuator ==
  note: Auxiliary diagnostic output vector: 1: valve opening 2: C1 pressure 3: C2 pressure 4: delta pressure 5: force 6: velocity 7: C1 flow 8: C2 flow 9: total flow 10: kinematic flow 11: compressibility flow 12: leakage flow 13: C1 oilspring displacement 14: C2 oilspring displacement 15: C1 oilspring velocity 16: C2 oilspring velocity
  note: Note: "1" and "2" denote actuator cylinders on either side of the actuator piston. With positive valve drive, oil is ported into cylinder 1, resulting in positive displacement.
  note: Parameter vector: 1: oil bulk modulus (force/displ^2) 2: servovalve delay (sec) 3: servovalve overlap 4: rated pressure (force/displ^2) 5: rated flow at rated pressure (displ^3/sec) 6: nominal flow at rated pressure (displ^3/sec) 7: actuator piston area 1 (displ^2) 8: actuator piston area 2 (displ^2) 9: actuator usable stroke 1 (displ) 10: actuator usable stroke 2 (displ) 11: actuator end cushion length 1 (displ) 12: actuator end cushion length 2 (displ) 13: additional port volume 1 (displ^3) 14: additional port volume 1 (displ^3) 15: actuator parasitic damping factor 16: cross-chamber leakage factor (flow/press) 17: ratio port openings according to area 18: sample period (sec) Conversion factors used for converting signals from external (user) to internal (canonical) units: 19: displacement 20: velocity 21: force 22: pressure 23: flow
  cmd : Inport
  displ : Inport  Port=2
  veloc : Inport  Port=3
  spl press : Inport  Port=4
  rtn press : Inport  Port=5
  abs : Abs  SaturateOnIntegerOverflow=on  SampleTime=-1
  actuator : S-Function  FunctionName=Actuator  Parameters=params
  total flow sel : Selector  InputType=Vector  ElementSrc=Internal  Elements=9  RowSrc=Internal  Rows=1  ColumnSrc=Internal  Columns=1  IndexIsStartValue=off
  force : Outport
  flow : Outport  Port=2
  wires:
  abs/1 -> flow/1
  total flow sel/1 -> abs/1
  actuator/2 -> total flow sel/1
  veloc/1 -> actuator/3
  displ/1 -> actuator/2
  actuator/1 -> force/1
  cmd/1 -> actuator/1
  rtn press/1 -> actuator/5
  spl press/1 -> actuator/4

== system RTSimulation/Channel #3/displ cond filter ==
  inp : Inport
  filter : DiscreteFilter  Numerator=b  Denominator=a  SampleTime=-1
  out : Outport
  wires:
  filter/1 -> out/1
  inp/1 -> filter/1

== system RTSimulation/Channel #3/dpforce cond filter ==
  inp : Inport
  filter : DiscreteFilter  Numerator=b  Denominator=a  SampleTime=-1
  out : Outport
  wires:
  inp/1 -> filter/1
  filter/1 -> out/1

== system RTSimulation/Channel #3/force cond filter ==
  inp : Inport
  filter : DiscreteFilter  Numerator=b  Denominator=a  SampleTime=-1
  out : Outport
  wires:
  filter/1 -> out/1
  inp/1 -> filter/1

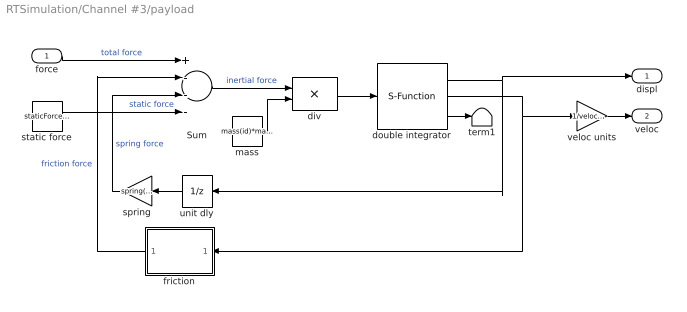
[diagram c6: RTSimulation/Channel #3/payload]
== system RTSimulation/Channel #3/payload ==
  force : Inport
  Sum : Sum  Inputs=+---
  div : Product  Inputs=*/
  double integrator : S-Function  FunctionName=doubleintegrator  Parameters=maxDispl, minDispl, initDispl, maxVeloc, minVeloc, initVeloc, samplePeriod  mask(Double integrator){maxDispl=maxDispl(id), minDispl=minDispl(id), initDispl=0, maxVeloc=maxVeloc(id)*velocCanon, minVeloc=minVeloc(id)*velocCanon, initVeloc=0, samplePeriod=samplePeriod}
      mask prompts: maxDispl "Maximum displacement"; minDispl "Minimum displacement"; initDispl "Initial displacement"; maxVeloc "Maximum velocity"; minVeloc "Minimum velocity"; initVeloc "Initial velocity"; samplePeriod "Sample period (sec)"
      mask help: Integrates acceleration twice to produce velocity and displacement. When clipping occurs, acceleration, velocity and displacement are adjusted accordingly.
  friction : Subsystem  Orientation=left  mask{friction=friction(id)*forceCanon, yieldDispl=yieldDispl(id)*lengthCanon, hysteresis=0}
      mask prompts: friction "Sliding friction"; yieldDispl "Equiv. yield displacement (in)"; hysteresis "Hysteresis constant"
  mass : Constant  Value=mass(id)*massCanon  OutDataType=sfix(16)  ConRadixGroup=Use specified scaling  OutScaling=2^0  SampleTime=inf  FramePeriod=inf
  spring : Gain  Orientation=left  Gain=spring(id)*springCanon
  static force : Constant  Value=staticForce(id)*forceCanon  OutDataType=sfix(16)  ConRadixGroup=Use specified scaling  OutScaling=2^0  SampleTime=inf  FramePeriod=inf
  term1 : Terminator
  unit dly : UnitDelay  Orientation=left  SampleTime=-1
  veloc units : Gain  Gain=1/velocCanon
  displ : Outport
  veloc : Outport  Port=2
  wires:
  double integrator/2 -> friction/1(veloc), veloc units/1
  double integrator/1 -> unit dly/1, displ/1
  div/1 -> double integrator/1
  double integrator/3 -> term1/1
  spring/1 -> Sum/3  "spring force"
  mass/1 -> div/2
  force/1 -> Sum/1  "total force"
  static force/1 -> Sum/4  "static force"
  Sum/1 -> div/1  "inertial force"
  veloc units/1 -> veloc/1
  unit dly/1 -> spring/1
  friction/1(force) -> Sum/2  "friction force"

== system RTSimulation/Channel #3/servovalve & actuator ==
  note: Parameter vector: 1: oil bulk modulus (force/displ^2) 2: servovalve delay (sec) 3: servovalve overlap 4: rated pressure (force/displ^2) 5: rated flow at rated pressure (displ^3/sec) 6: nominal flow at rated pressure (displ^3/sec) 7: actuator piston area 1 (displ^2) 8: actuator piston area 2 (displ^2) 9: actuator usable stroke 1 (displ) 10: actuator usable stroke 2 (displ) 11: actuator end cushion length 1 (displ) 12: actuator end cushion length 2 (displ) 13: additional port volume 1 (displ^3) 14: additional port volume 1 (displ^3) 15: actuator parasitic damping factor 16: cross-chamber leakage factor (flow/press) 17: ratio port openings according to area 18: sample period (sec) Conversion factors used for converting signals from external (user) to internal (canonical) units: 19: displacement 20: velocity 21: force 22: pressure 23: flow
  note: Note: "1" and "2" denote actuator cylinders on either side of the actuator piston. With positive valve drive, oil is ported into cylinder 1, resulting in positive displacement.
  note: Auxiliary diagnostic output vector: 1: valve opening 2: C1 pressure 3: C2 pressure 4: delta pressure 5: force 6: velocity 7: C1 flow 8: C2 flow 9: total flow 10: kinematic flow 11: compressibility flow 12: leakage flow 13: C1 oilspring displacement 14: C2 oilspring displacement 15: C1 oilspring velocity 16: C2 oilspring velocity
  cmd : Inport
  displ : Inport  Port=2
  veloc : Inport  Port=3
  spl press : Inport  Port=4
  rtn press : Inport  Port=5
  abs : Abs  SaturateOnIntegerOverflow=on  SampleTime=-1
  actuator : S-Function  FunctionName=Actuator  Parameters=params
  total flow sel : Selector  InputType=Vector  ElementSrc=Internal  Elements=9  RowSrc=Internal  Rows=1  ColumnSrc=Internal  Columns=1  IndexIsStartValue=off
  force : Outport
  flow : Outport  Port=2
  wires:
  spl press/1 -> actuator/4
  rtn press/1 -> actuator/5
  cmd/1 -> actuator/1
  actuator/1 -> force/1
  displ/1 -> actuator/2
  veloc/1 -> actuator/3
  actuator/2 -> total flow sel/1
  total flow sel/1 -> abs/1
  abs/1 -> flow/1

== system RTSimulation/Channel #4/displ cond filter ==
  inp : Inport
  filter : DiscreteFilter  Numerator=b  Denominator=a  SampleTime=-1
  out : Outport
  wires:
  inp/1 -> filter/1
  filter/1 -> out/1

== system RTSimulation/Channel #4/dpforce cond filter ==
  inp : Inport
  filter : DiscreteFilter  Numerator=b  Denominator=a  SampleTime=-1
  out : Outport
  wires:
  filter/1 -> out/1
  inp/1 -> filter/1

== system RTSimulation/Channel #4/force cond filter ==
  inp : Inport
  filter : DiscreteFilter  Numerator=b  Denominator=a  SampleTime=-1
  out : Outport
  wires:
  inp/1 -> filter/1
  filter/1 -> out/1

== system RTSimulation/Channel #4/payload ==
  force : Inport
  Sum : Sum  Inputs=+---
  div : Product  Inputs=*/
  double integrator : S-Function  FunctionName=doubleintegrator  Parameters=maxDispl, minDispl, initDispl, maxVeloc, minVeloc, initVeloc, samplePeriod  mask(Double integrator){maxDispl=maxDispl(id), minDispl=minDispl(id), initDispl=0, maxVeloc=maxVeloc(id)*velocCanon, minVeloc=minVeloc(id)*velocCanon, initVeloc=0, samplePeriod=samplePeriod}
      mask prompts: maxDispl "Maximum displacement"; minDispl "Minimum displacement"; initDispl "Initial displacement"; maxVeloc "Maximum velocity"; minVeloc "Minimum velocity"; initVeloc "Initial velocity"; samplePeriod "Sample period (sec)"
      mask help: Integrates acceleration twice to produce velocity and displacement. When clipping occurs, acceleration, velocity and displacement are adjusted accordingly.
  friction : Subsystem  Orientation=left  mask{friction=friction(id)*forceCanon, yieldDispl=yieldDispl(id)*lengthCanon, hysteresis=0}
      mask prompts: friction "Sliding friction"; yieldDispl "Equiv. yield displacement (in)"; hysteresis "Hysteresis constant"
  mass : Constant  Value=mass(id)*massCanon  OutDataType=sfix(16)  ConRadixGroup=Use specified scaling  OutScaling=2^0  SampleTime=inf  FramePeriod=inf
  spring : Gain  Orientation=left  Gain=spring(id)*springCanon
  static force : Constant  Value=staticForce(id)*forceCanon  OutDataType=sfix(16)  ConRadixGroup=Use specified scaling  OutScaling=2^0  SampleTime=inf  FramePeriod=inf
  term1 : Terminator
  unit dly : UnitDelay  Orientation=left  SampleTime=-1
  veloc units : Gain  Gain=1/velocCanon
  displ : Outport
  veloc : Outport  Port=2
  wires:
  friction/1(force) -> Sum/2  "friction force"
  unit dly/1 -> spring/1
  veloc units/1 -> veloc/1
  Sum/1 -> div/1  "inertial force"
  static force/1 -> Sum/4  "static force"
  force/1 -> Sum/1  "total force"
  mass/1 -> div/2
  spring/1 -> Sum/3  "spring force"
  double integrator/3 -> term1/1
  div/1 -> double integrator/1
  double integrator/1 -> displ/1, unit dly/1
  double integrator/2 -> veloc units/1, friction/1(veloc)

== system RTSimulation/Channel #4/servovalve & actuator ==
  note: Auxiliary diagnostic output vector: 1: valve opening 2: C1 pressure 3: C2 pressure 4: delta pressure 5: force 6: velocity 7: C1 flow 8: C2 flow 9: total flow 10: kinematic flow 11: compressibility flow 12: leakage flow 13: C1 oilspring displacement 14: C2 oilspring displacement 15: C1 oilspring velocity 16: C2 oilspring velocity
  note: Note: "1" and "2" denote actuator cylinders on either side of the actuator piston. With positive valve drive, oil is ported into cylinder 1, resulting in positive displacement.
  note: Parameter vector: 1: oil bulk modulus (force/displ^2) 2: servovalve delay (sec) 3: servovalve overlap 4: rated pressure (force/displ^2) 5: rated flow at rated pressure (displ^3/sec) 6: nominal flow at rated pressure (displ^3/sec) 7: actuator piston area 1 (displ^2) 8: actuator piston area 2 (displ^2) 9: actuator usable stroke 1 (displ) 10: actuator usable stroke 2 (displ) 11: actuator end cushion length 1 (displ) 12: actuator end cushion length 2 (displ) 13: additional port volume 1 (displ^3) 14: additional port volume 1 (displ^3) 15: actuator parasitic damping factor 16: cross-chamber leakage factor (flow/press) 17: ratio port openings according to area 18: sample period (sec) Conversion factors used for converting signals from external (user) to internal (canonical) units: 19: displacement 20: velocity 21: force 22: pressure 23: flow
  cmd : Inport
  displ : Inport  Port=2
  veloc : Inport  Port=3
  spl press : Inport  Port=4
  rtn press : Inport  Port=5
  abs : Abs  SaturateOnIntegerOverflow=on  SampleTime=-1
  actuator : S-Function  FunctionName=Actuator  Parameters=params
  total flow sel : Selector  InputType=Vector  ElementSrc=Internal  Elements=9  RowSrc=Internal  Rows=1  ColumnSrc=Internal  Columns=1  IndexIsStartValue=off
  force : Outport
  flow : Outport  Port=2
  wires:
  abs/1 -> flow/1
  total flow sel/1 -> abs/1
  actuator/2 -> total flow sel/1
  veloc/1 -> actuator/3
  displ/1 -> actuator/2
  actuator/1 -> force/1
  cmd/1 -> actuator/1
  rtn press/1 -> actuator/5
  spl press/1 -> actuator/4

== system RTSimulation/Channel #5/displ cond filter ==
  inp : Inport
  filter : DiscreteFilter  Numerator=b  Denominator=a  SampleTime=-1
  out : Outport
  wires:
  filter/1 -> out/1
  inp/1 -> filter/1

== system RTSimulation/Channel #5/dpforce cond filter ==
  inp : Inport
  filter : DiscreteFilter  Numerator=b  Denominator=a  SampleTime=-1
  out : Outport
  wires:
  inp/1 -> filter/1
  filter/1 -> out/1

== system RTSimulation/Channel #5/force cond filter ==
  inp : Inport
  filter : DiscreteFilter  Numerator=b  Denominator=a  SampleTime=-1
  out : Outport
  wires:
  filter/1 -> out/1
  inp/1 -> filter/1

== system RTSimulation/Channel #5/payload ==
  force : Inport
  Sum : Sum  Inputs=+---
  div : Product  Inputs=*/
  double integrator : S-Function  FunctionName=doubleintegrator  Parameters=maxDispl, minDispl, initDispl, maxVeloc, minVeloc, initVeloc, samplePeriod  mask(Double integrator){maxDispl=maxDispl(id), minDispl=minDispl(id), initDispl=0, maxVeloc=maxVeloc(id)*velocCanon, minVeloc=minVeloc(id)*velocCanon, initVeloc=0, samplePeriod=samplePeriod}
      mask prompts: maxDispl "Maximum displacement"; minDispl "Minimum displacement"; initDispl "Initial displacement"; maxVeloc "Maximum velocity"; minVeloc "Minimum velocity"; initVeloc "Initial velocity"; samplePeriod "Sample period (sec)"
      mask help: Integrates acceleration twice to produce velocity and displacement. When clipping occurs, acceleration, velocity and displacement are adjusted accordingly.
  friction : Subsystem  Orientation=left  mask{friction=friction(id)*forceCanon, yieldDispl=yieldDispl(id)*lengthCanon, hysteresis=0}
      mask prompts: friction "Sliding friction"; yieldDispl "Equiv. yield displacement (in)"; hysteresis "Hysteresis constant"
  mass : Constant  Value=mass(id)*massCanon  OutDataType=sfix(16)  ConRadixGroup=Use specified scaling  OutScaling=2^0  SampleTime=inf  FramePeriod=inf
  spring : Gain  Orientation=left  Gain=spring(id)*springCanon
  static force : Constant  Value=staticForce(id)*forceCanon  OutDataType=sfix(16)  ConRadixGroup=Use specified scaling  OutScaling=2^0  SampleTime=inf  FramePeriod=inf
  term1 : Terminator
  unit dly : UnitDelay  Orientation=left  SampleTime=-1
  veloc units : Gain  Gain=1/velocCanon
  displ : Outport
  veloc : Outport  Port=2
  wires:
  double integrator/2 -> friction/1(veloc), veloc units/1
  double integrator/1 -> unit dly/1, displ/1
  div/1 -> double integrator/1
  double integrator/3 -> term1/1
  spring/1 -> Sum/3  "spring force"
  mass/1 -> div/2
  force/1 -> Sum/1  "total force"
  static force/1 -> Sum/4  "static force"
  Sum/1 -> div/1  "inertial force"
  veloc units/1 -> veloc/1
  unit dly/1 -> spring/1
  friction/1(force) -> Sum/2  "friction force"
